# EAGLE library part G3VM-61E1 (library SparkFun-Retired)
Omron NO solid state relay
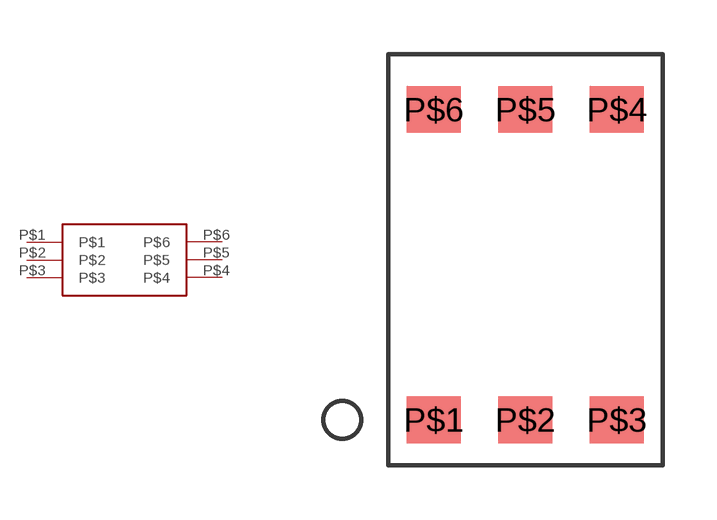
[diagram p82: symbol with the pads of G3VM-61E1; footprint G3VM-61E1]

Designator prefix -

## G3VM-61E1 (PROD_ID: TRANS-08720)  [G3VM-61E1]
P$1  P$1
P$2  P$2
P$3  P$3
P$4  P$4
P$5  P$5
P$6  P$6

## Footprint G3VM-61E1 (pad centres in mm)
smd 1.5 x 1.3: P$1 0,0; P$2 2.54,0; P$3 5.08,0; P$4 5.08,8.62; P$5 2.54,8.62; P$6 0,8.62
